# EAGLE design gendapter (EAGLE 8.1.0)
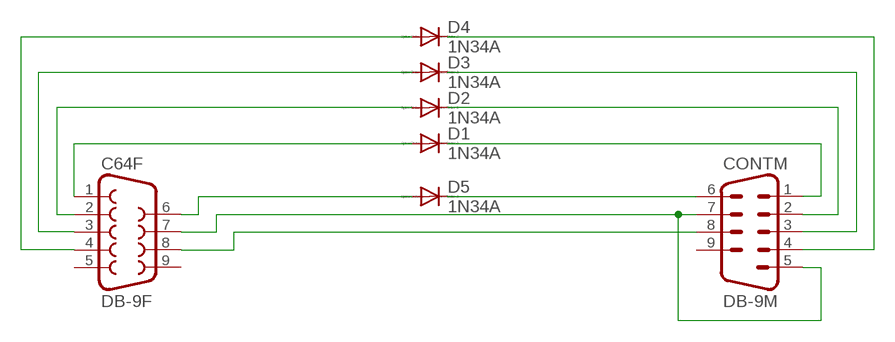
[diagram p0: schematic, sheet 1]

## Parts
C64F  DB-9F  F09D  [F09D]
CONTM  DB-9M  M09D  [M09D]
D1  1N34A  DIODE-DO35-10  [DO35-10]
D2  1N34A  DIODE-DO35-10  [DO35-10]
D3  1N34A  DIODE-DO35-10  [DO35-10]
D4  1N34A  DIODE-DO35-10  [DO35-10]
D5  1N34A  DIODE-DO35-10  [DO35-10]

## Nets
N$1: C64F.1 D1.A
N$2: CONTM.1 D1.C
N$3: CONTM.2 D2.C
N$4: C64F.2 D2.A
N$5: C64F.3 D3.A
N$6: CONTM.3 D3.C
N$7: C64F.4 D4.A
N$8: CONTM.4 D4.C
N$9: C64F.6 D5.A
N$10: CONTM.6 D5.C
N$11: C64F.7 CONTM.5 CONTM.7
N$12: C64F.8 CONTM.8
Unconnected: C64F.5 C64F.9 CONTM.9

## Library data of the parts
C64F = con-subd:F09: SUB-D; OC_FARNELL: unknown; OC_NEWARK: unknown
CONTM = con-subd:M09: SUB-D; OC_FARNELL: unknown; OC_NEWARK: unknown
D1-D5 = diode:DIODE-: DIODE

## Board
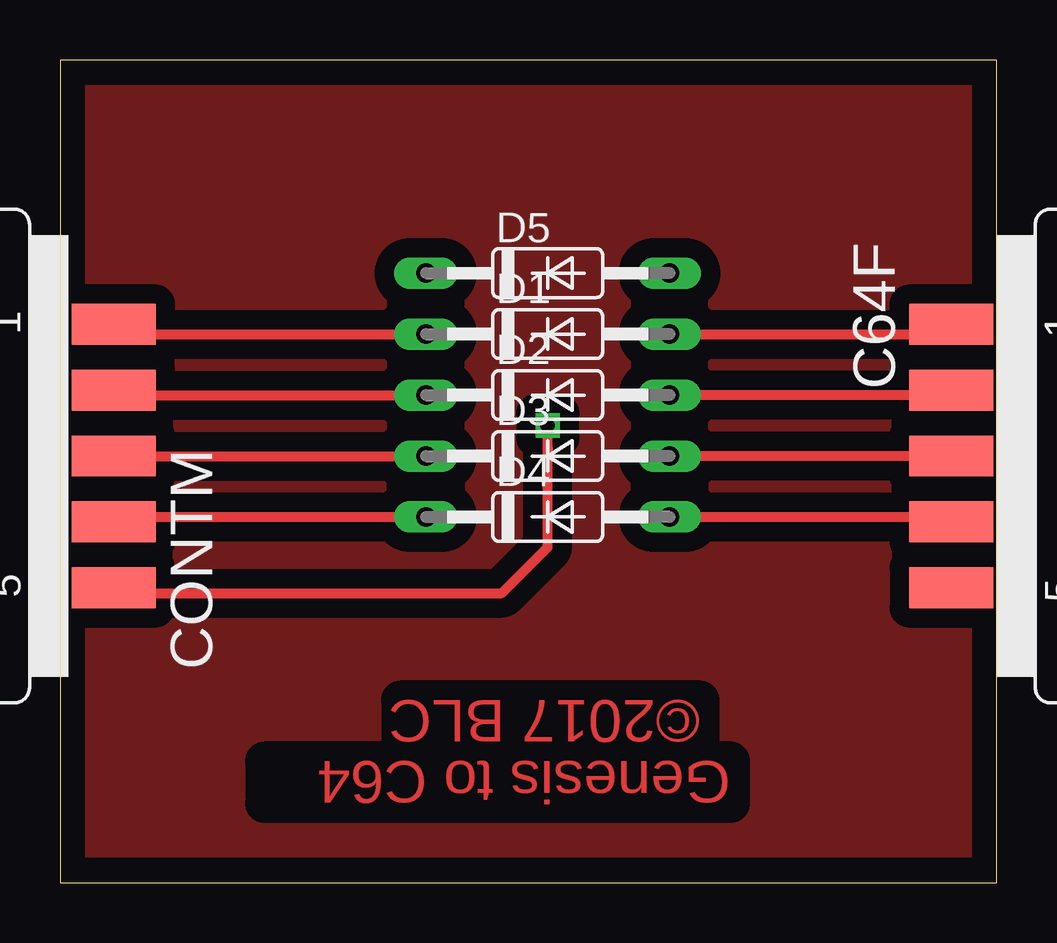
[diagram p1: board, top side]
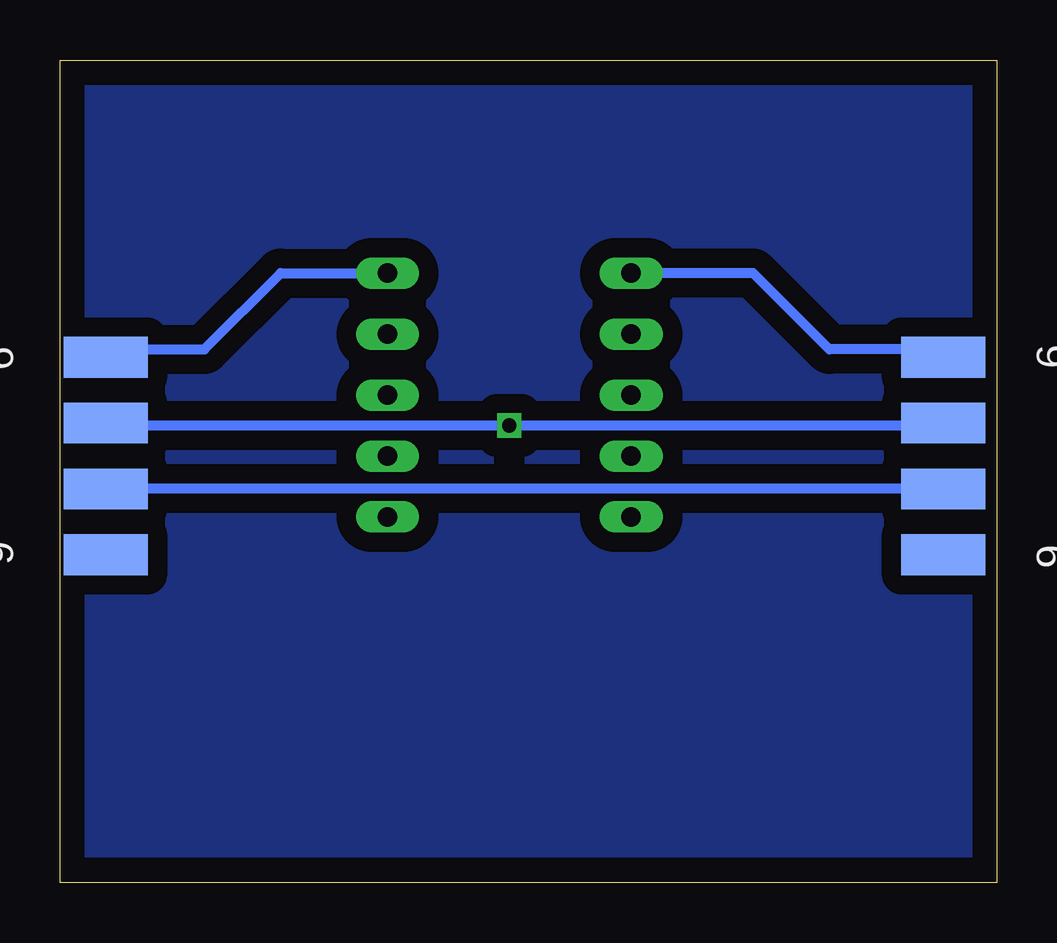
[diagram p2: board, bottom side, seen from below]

Size 39.04 x 34.28 mm. Coordinates in mm from the lower left corner, seen from the top.
Outline: 0,0 39.04,0 39.04,34.28 0,34.28 0,0
Copper layers (1*16): Top 0.035mm / dielectric 1.5mm / Bottom 0.035mm
Design rules "default": minimum track width 10mil, minimum drill 24mil, track to track 8mil, track to pad 8mil, pad to pad 8mil, via to via 8mil, smd to smd 8mil, copper to edge 40mil, drill to drill 8mil, minimum pad ring 10mil, minimum via ring 8mil, stop-mask expansion 4mil, vias tented up to drill 0mil, thermal gap 10mil

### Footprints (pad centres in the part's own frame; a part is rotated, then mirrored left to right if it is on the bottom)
F09D = smd 1.7 x 3.5: 1 -5.486,-6.045; 2 -2.743,-6.045; 3 0,-6.045; 4 2.743,-6.045; 5 5.486,-6.045 | smd 1.7 x 3.5 bottom: 6 -4.115,-6.045; 7 -1.372,-6.045; 8 1.372,-6.045; 9 4.115,-6.045
M09D = smd 1.7 x 3.5: 1 5.486,-6.045; 2 2.743,-6.045; 3 0,-6.045; 4 -2.743,-6.045; 5 -5.486,-6.045 | smd 1.7 x 3.5 bottom: 6 4.115,-6.045; 7 1.372,-6.045; 8 -1.372,-6.045; 9 -4.115,-6.045
DO35-10 = drill 0.813 long: A 5.08,0; C -5.08,0

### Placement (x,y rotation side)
C64F  43.18,17.78 270 top
CONTM  -3.81,17.78 90 top
D1  20.32,22.86 0 top
D2  20.32,20.32 0 top
D3  20.32,17.78 0 top
D4  20.32,15.24 0 top
D5  20.32,25.4 0 top

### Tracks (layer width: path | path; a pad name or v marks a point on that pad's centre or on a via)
GND
  pour Top (isolate 0.813): 0,1.27 39.37,1.27 39.37,33.02 0,33.02
  pour Bottom (isolate 0.813): 0,33.02 39.37,33.02 39.37,1.27 0,1.27
N$1
  Top 0.254: 36.85,22.99 37.08,23.22 C64F.1
  Top 0.406: D1.A 35.56,22.86 35.97,23.27 C64F.1
N$2
  Top 0.254: 2.56,22.99 2.34,23.22 CONTM.1
  Top 0.406: CONTM.1 2.64,22.86 D1.C
N$3
  Top 0.254: 2.34,20.47 CONTM.2
  Top 0.406: CONTM.2 2.44,20.32 D2.C
N$4
  Top 0.254: 37.08,20.47 C64F.2
  Top 0.406: C64F.2 36.93,20.32 D2.A
N$5
  Top 0.254: 37.08,17.96 C64F.3
  Top 0.406: C64F.3 D3.A
N$6
  Top 0.254: 2.34,17.96 CONTM.3
  Top 0.406: CONTM.3 D3.C
N$7
  Top 0.254: C64F.4 37.08,14.99
  Top 0.406: C64F.4 35.76,15.04 35.56,15.24 D4.A
N$8
  Top 0.254: 2.34,14.99 CONTM.4
  Top 0.406: CONTM.4 2.44,15.24 D4.C
N$9
  Bottom 0.254: 37.08,22.07 C64F.6
  Bottom 0.406: C64F.6 36.8,22.22 33.02,22.22 29.84,25.4 D5.A
N$10
  Bottom 0.254: 2.34,22.07 CONTM.6
  Bottom 0.406: CONTM.6 2.56,22.22 6.98,22.22 10.16,25.4 D5.C
N$11  (via drill 0.6)
  Top 0.254: 1.65,12.47 2.11,12.47 CONTM.5
  Top 0.406: CONTM.5 2.46,12.06 18.41,12.06 20.32,13.97 20.32,17.78 | 20.32,17.78 20.32,18.14 20.32,17.78 | 20.32,17.78 v20.32,19.05
  Bottom 0.254: C64F.7 37.08,19.33 | 2.34,19.33 CONTM.7
  Bottom 0.406: CONTM.7 2.34,19.05 v20.32,19.05 35.56,19.05 35.66,19.15 C64F.7
N$12
  Bottom 0.254: 2.34,16.59 CONTM.8 | C64F.8 37.08,16.59
  Bottom 0.406: CONTM.8 C64F.8

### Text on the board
Top: ©2017 BLC | Genesis to C64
